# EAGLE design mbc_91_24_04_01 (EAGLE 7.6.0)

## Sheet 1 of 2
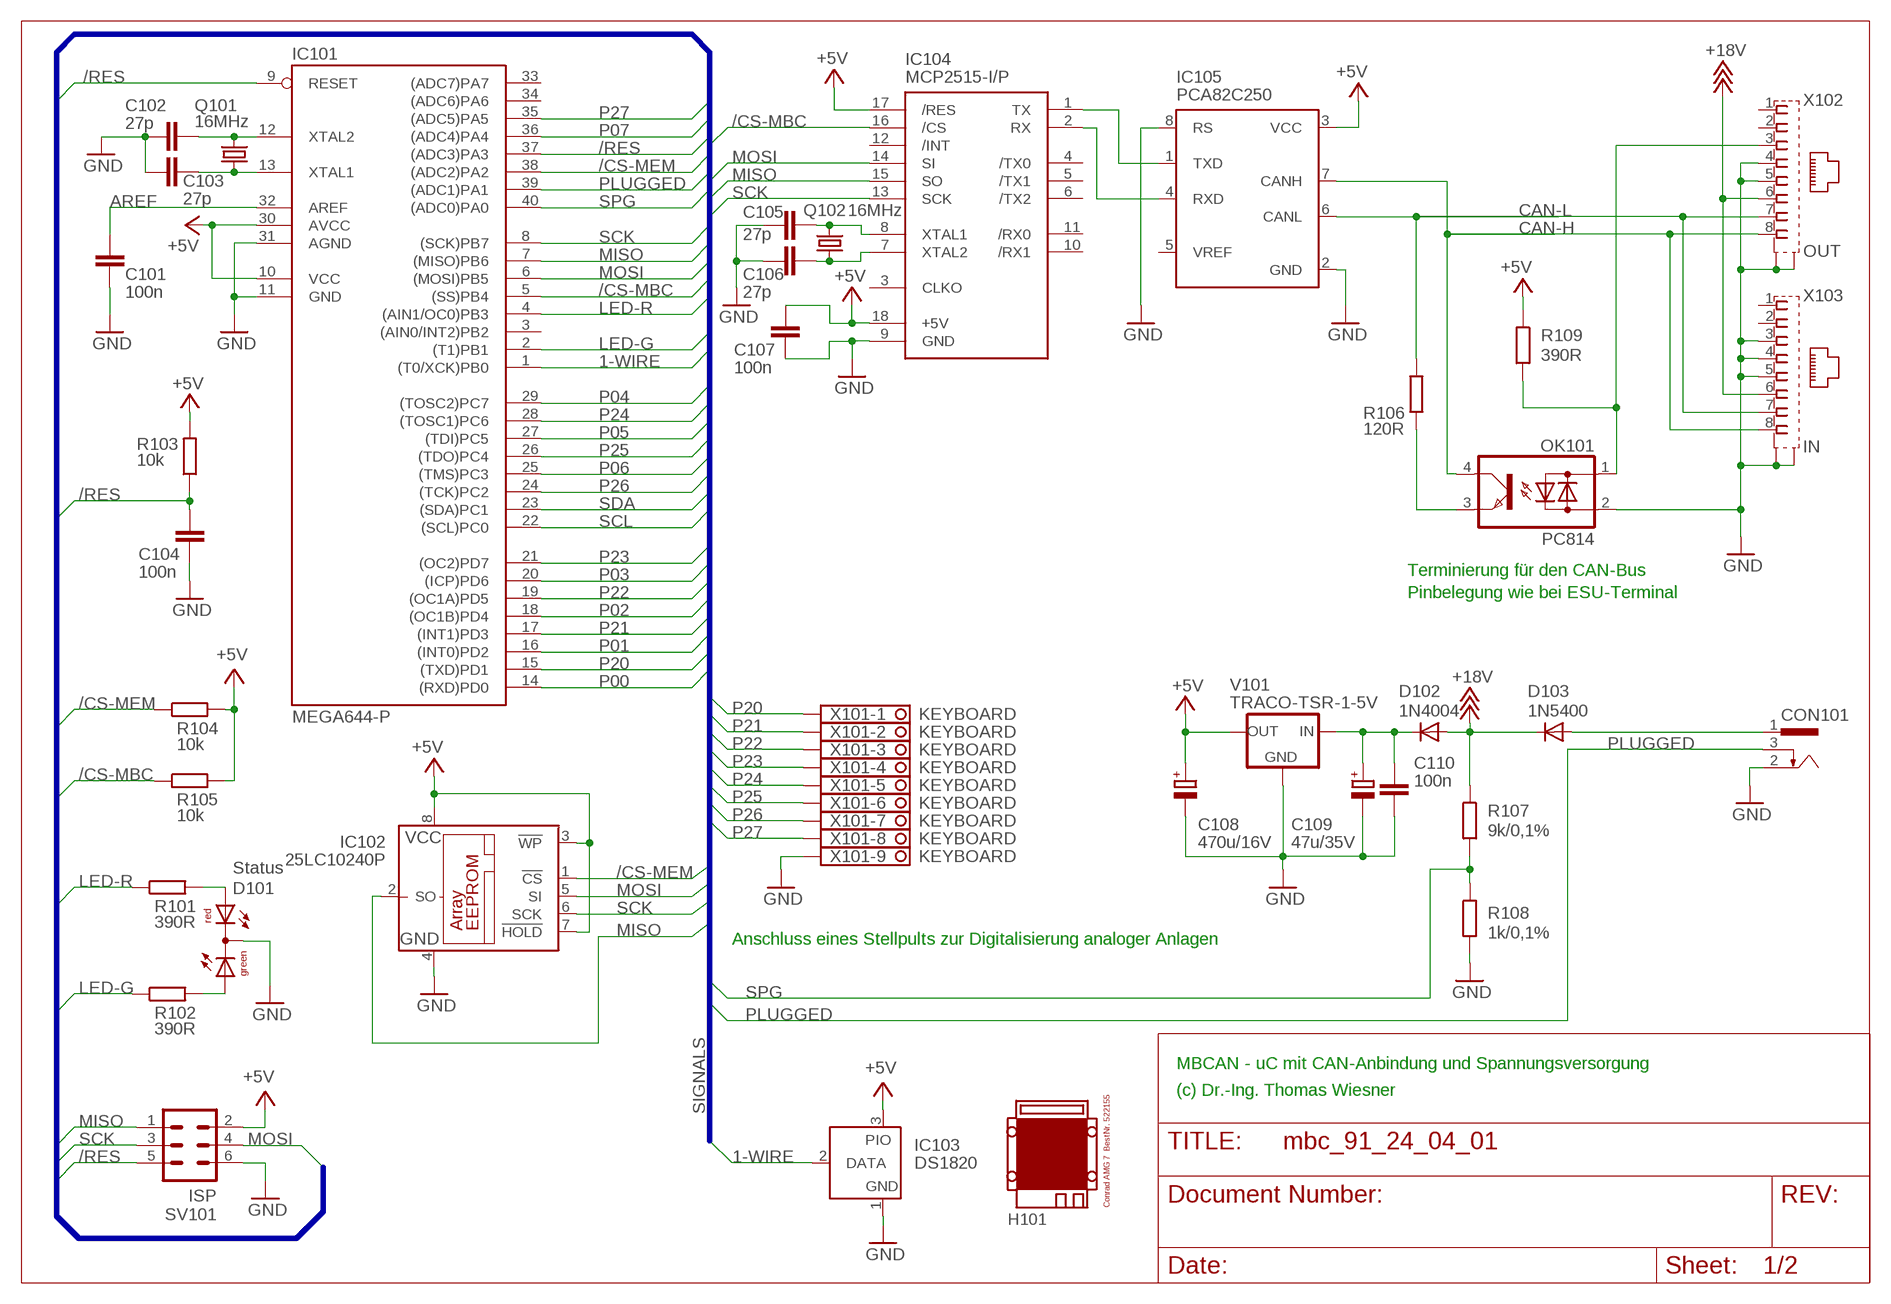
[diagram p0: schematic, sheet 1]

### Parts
C101  100n  C-EU025-025X050  [C025-025X050]
C102  27p  C-EU025-025X050  [C025-025X050]
C103  27p  C-EU025-025X050  [C025-025X050]
C104  100n  C-EU025-025X050  [C025-025X050]
C105  27p  C-EU025-025X050  [C025-025X050]
C106  27p  C-EU025-025X050  [C025-025X050]
C107  100n  C-EU025-025X050  [C025-025X050]
C108  470u/16V  CPOL-EUE3.5-8  [E3,5-8]
C109  47u/35V  CPOL-EUE2.5-7  [E2,5-7]
C110  100n  C-EU025-025X050  [C025-025X050]
CON101  POWER-JACK  [POWER-JACK]
D101  Status  DUOLED5MM  [DUOLED5MM]
D102  1N4004  [DO41-10]
D103  1N5400  [DO201-15]
H101  MODULGEHÄUSE-AMG-7  [MODULGEHÄUSE-AMG-7]
IC101  MEGA644-P  MEGA323-P  [DIL40]
IC102  25LC10240P  25LC040P  [DIL8]
IC103  DS1820  DS2405  [TO92-]
IC104  MCP2515-I/P  MCP2510-I/P  [DIL18]
IC105  PCA82C250  [DIL08]
OK101  PC814  [DIL04]
Q101  16MHz  CRYSTALHC49U70  [HC49U70]
Q102  16MHz  CRYSTALHC49U70  [HC49U70]
R101  390R  R-EU_0207/10  [0207/10]
R102  390R  R-EU_0207/10  [0207/10]
R103  10k  R-EU_0207/10  [0207/10]
R104  10k  R-EU_0207/10  [0207/10]
R105  10k  R-EU_0207/10  [0207/10]
R106  120R  R-EU_0207/10  [0207/10]
R107  9k/0,1%  R-EU_0207/10  [0207/10]
R108  1k/0,1%  R-EU_0207/10  [0207/10]
R109  390R  R-EU_0207/10  [0207/10]
SV101  ISP  ML6  [ML6]
V101  TRACO-TSR-1-5V  [TRACO-TSR-1]
X101  KEYBOARD  1751316  [1751316]
X102  OUT  0446200002  [0446200002]
X103  IN  0446200002  [0446200002]

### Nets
1-WIRE: IC101.1((T0/XCK)PB0) IC103.2(DATA)
+5V: C107.1 C108.+ IC101.10(VCC) IC101.30(AVCC) IC102.3(!WP) IC102.7(!HOLD) IC102.8(VCC) IC103.3(PIO) IC104.17(/RES) IC104.18(+5V) IC105.3(VCC) R103.2 R104.2 R105.2 R109.1 SV101.2 V101.OUT ; also sheet 2
+18V: D102.A D103.C R107.1 X102.6 X103.6 ; also sheet 2
/CS-MBC: IC101.5((SS)PB4) IC104.16(/CS) R105.1
/CS-MEM: IC101.38((ADC2)PA2) IC102.1(!CS) R104.1
/RES: C104.1 IC101.9(RESET) IC101.37((ADC3)PA3) R103.1 SV101.5
AREF: C101.1 IC101.32(AREF)
CAN-H: IC105.7(CANH) OK101.4(C) X102.8 X103.8
CAN-L: IC105.6(CANL) R106.2 X102.7 X103.7
GND: C101.2 C102.1 C103.1 C104.2 C105.1 C106.1 C107.2 C108.- C109.- C110.2 CON101.2 D101.K(C) IC101.11(GND) IC101.31(AGND) IC102.4(GND) IC103.1(GND) IC104.9(GND) IC105.2(GND) IC105.8(RS) OK101.2(AC2) R108.2 SV101.6 V101.GND X101.9 X102.4 X102.5 X102.S@1(S1) X102.S@2(S2) X103.3 X103.4 X103.5 X103.S@1(S1) X103.S@2(S2) ; also sheet 2
LED-G: IC101.2((T1)PB1) R102.1
LED-R: IC101.4((AIN1/OC0)PB3) R101.1
MISO: IC101.7((MISO)PB6) IC102.2(SO) IC104.15(SO) SV101.1
MOSI: IC101.6((MOSI)PB5) IC102.5(SI) IC104.14(SI) SV101.4
N$1: IC104.1(TX) IC105.1(TXD)
N$2: IC104.2(RX) IC105.4(RXD)
N$3: OK101.3(E) R106.1
N$4: OK101.1(AC1) R109.2 X102.3
N$6: C109.+ C110.1 D102.C V101.IN
N$9: D101.AR R101.2
N$13: D101.AG R102.2
N$21: C102.2 IC101.12(XTAL2) Q101.2
N$22: C103.2 IC101.13(XTAL1) Q101.1
N$23: C105.2 IC104.8(XTAL1) Q102.2
N$24: C106.2 IC104.7(XTAL2) Q102.1
P00: IC101.14((RXD)PD0) ; also sheet 2
P01: IC101.16((INT0)PD2) ; also sheet 2
P02: IC101.18((OC1B)PD4) ; also sheet 2
P03: IC101.20((ICP)PD6) ; also sheet 2
P04: IC101.29((TOSC2)PC7) ; also sheet 2
P05: IC101.27((TDI)PC5) ; also sheet 2
P06: IC101.25((TMS)PC3) ; also sheet 2
P07: IC101.36((ADC4)PA4) ; also sheet 2
P20: IC101.15((TXD)PD1) X101.1
P21: IC101.17((INT1)PD3) X101.2
P22: IC101.19((OC1A)PD5) X101.3
P23: IC101.21((OC2)PD7) X101.4
P24: IC101.28((TOSC1)PC6) X101.5
P25: IC101.26((TDO)PC4) X101.6
P26: IC101.24((TCK)PC2) X101.7
P27: IC101.35((ADC5)PA5) X101.8
PLUGGED: CON101.3 IC101.39((ADC1)PA1)
SCK: IC101.8((SCK)PB7) IC102.6(SCK) IC104.13(SCK) SV101.3
SCL: IC101.22((SCL)PC0) ; also sheet 2
SDA: IC101.23((SDA)PC1) ; also sheet 2
SPG: IC101.40((ADC0)PA0) R107.2 R108.1
V-NETZTEIL: CON101.1 D103.A
Unconnected: IC101.3((AIN0/INT2)PB2) IC101.33((ADC7)PA7) IC101.34((ADC6)PA6) IC104.3(CLKO) IC104.4(/TX0) IC104.5(/TX1) IC104.6(/TX2) IC104.10(/RX1) IC104.11(/RX0) IC104.12(/INT) IC105.5(VREF) X102.1 X102.2 X103.1 X103.2

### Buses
SIGNALS

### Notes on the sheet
- Terminierung für den CAN-Bus
- Pinbelegung wie bei ESU-Terminal
- Anschluss eines Stellpults zur Digitalisierung analoger Anlagen
- MBCAN - uC mit CAN-Anbindung und Spannungsversorgung
- (c) Dr.-Ing. Thomas Wiesner

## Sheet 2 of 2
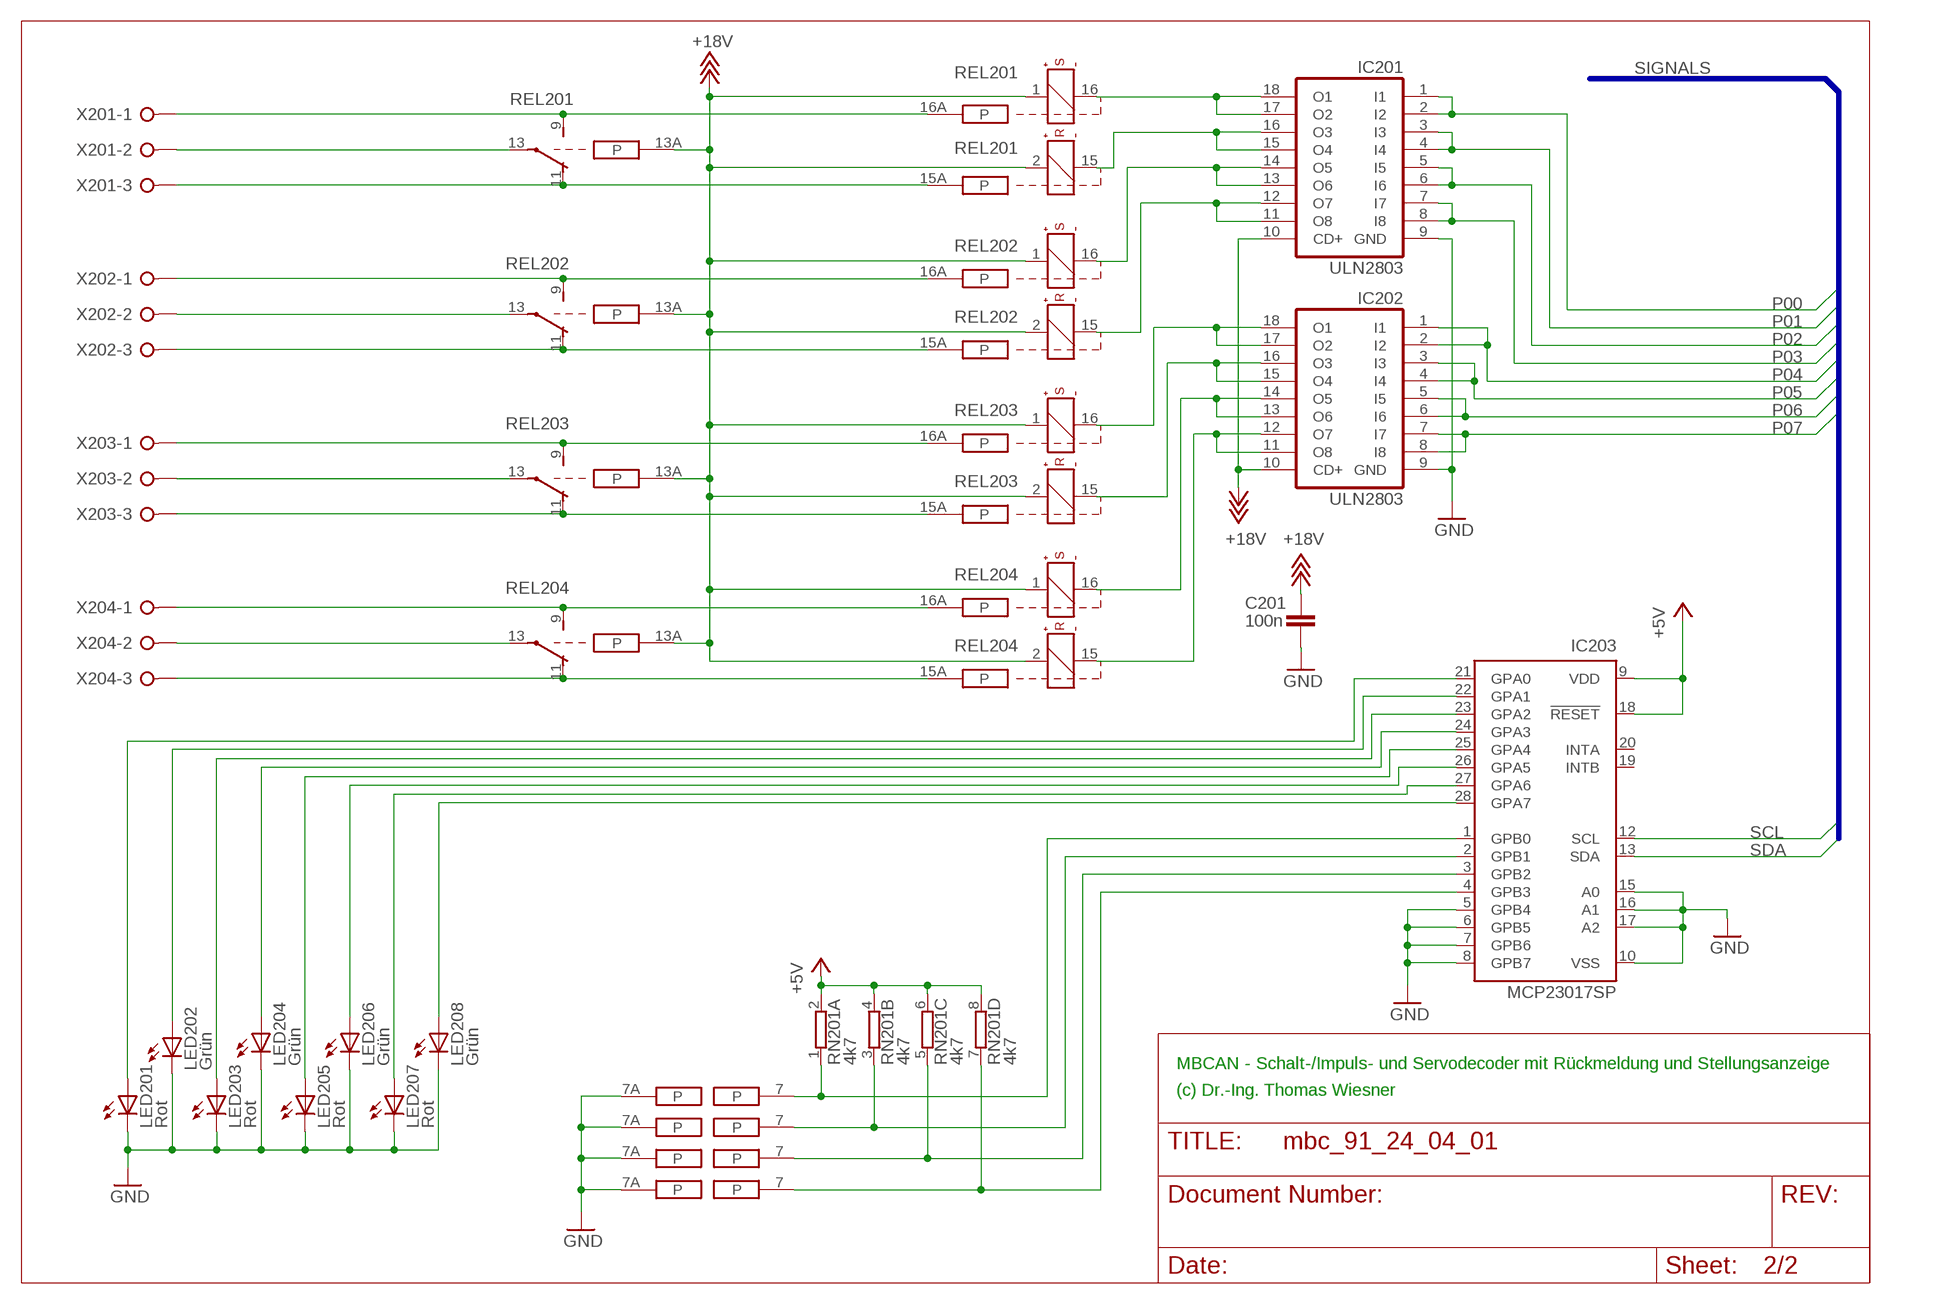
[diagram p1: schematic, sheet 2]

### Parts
C201  100n  C-EU025-025X050  [C025-025X050]
IC201  ULN2803  ULN2803A  [DIL18]
IC202  ULN2803  ULN2803A  [DIL18]
IC203  MCP23017SP  [DIL28-3]
LED201  Rot  LED3MM  [LED3MM]
LED202  Grün  LED3MM  [LED3MM]
LED203  Rot  LED3MM  [LED3MM]
LED204  Grün  LED3MM  [LED3MM]
LED205  Rot  LED3MM  [LED3MM]
LED206  Grün  LED3MM  [LED3MM]
LED207  Rot  LED3MM  [LED3MM]
LED208  Grün  LED3MM  [LED3MM]
REL201  RELAIS+PADS  [REL-BIPOLAR-LOETPADS]
REL202  RELAIS+PADS  [REL-BIPOLAR-LOETPADS]
REL203  RELAIS+PADS  [REL-BIPOLAR-LOETPADS]
REL204  RELAIS+PADS  [REL-BIPOLAR-LOETPADS]
RN201  4k7  E4R  [SIL8]
X201  W237-03P  [W237-133]
X202  W237-03P  [W237-133]
X203  W237-03P  [W237-133]
X204  W237-03P  [W237-133]

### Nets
+5V: IC203.9(VDD) IC203.18(!RESET) RN201.2 RN201.4 RN201.6 RN201.8 ; also sheet 1
+18V: C201.1 IC201.10(CD+) IC202.10(CD+) REL201.1(+) REL201.2(+) REL201.13A(P) REL202.1(+) REL202.2(+) REL202.13A(P) REL203.1(+) REL203.2(+) REL203.13A(P) REL204.1(+) REL204.2(+) REL204.13A(P) ; also sheet 1
GND: C201.2 IC201.9(GND) IC202.9(GND) IC203.5(GPB4) IC203.6(GPB5) IC203.7(GPB6) IC203.8(GPB7) IC203.10(VSS) IC203.15(A0) IC203.16(A1) IC203.17(A2) LED201.K(C) LED202.K(C) LED203.K(C) LED204.K(C) LED205.K(C) LED206.K(C) LED207.K(C) LED208.K(C) REL201.7A(P) REL202.7A(P) REL203.7A(P) REL204.7A(P) ; also sheet 1
K11: REL201.9(S) REL201.16A(P) X201.1
K12: REL201.13(P) X201.2
K13: REL201.11(O) REL201.15A(P) X201.3
K21: REL202.9(S) REL202.16A(P) X202.1
K22: REL202.13(P) X202.2
K23: REL202.11(O) REL202.15A(P) X202.3
K31: REL203.9(S) REL203.16A(P) X203.1
K32: REL203.13(P) X203.2
K33: REL203.11(O) REL203.15A(P) X203.3
K41: REL204.9(S) REL204.16A(P) X204.1
K42: REL204.13(P) X204.2
K43: REL204.11(O) REL204.15A(P) X204.3
N$5: IC203.22(GPA1) LED202.A
N$7: IC203.21(GPA0) LED201.A
N$8: IC201.15(O4) IC201.16(O3) REL201.15(-)
N$10: IC203.23(GPA2) LED203.A
N$11: IC203.25(GPA4) LED205.A
N$12: IC203.27(GPA6) LED207.A
N$14: IC203.1(GPB0) REL201.7(P) RN201.1
N$15: IC203.2(GPB1) REL202.7(P) RN201.3
N$16: IC203.3(GPB2) REL203.7(P) RN201.5
N$17: IC203.4(GPB3) REL204.7(P) RN201.7
N$18: IC203.24(GPA3) LED204.A
N$19: IC203.26(GPA5) LED206.A
N$20: IC203.28(GPA7) LED208.A
N$37: IC201.11(O8) IC201.12(O7) REL202.15(-)
N$50: IC202.15(O4) IC202.16(O3) REL203.15(-)
N$52: IC202.11(O8) IC202.12(O7) REL204.15(-)
P00: IC201.1(I1) IC201.2(I2) ; also sheet 1
P01: IC201.3(I3) IC201.4(I4) ; also sheet 1
P02: IC201.5(I5) IC201.6(I6) ; also sheet 1
P03: IC201.7(I7) IC201.8(I8) ; also sheet 1
P04: IC202.1(I1) IC202.2(I2) ; also sheet 1
P05: IC202.3(I3) IC202.4(I4) ; also sheet 1
P06: IC202.5(I5) IC202.6(I6) ; also sheet 1
P07: IC202.7(I7) IC202.8(I8) ; also sheet 1
S1: IC201.17(O2) IC201.18(O1) REL201.16(-)
S2: IC201.13(O6) IC201.14(O5) REL202.16(-)
S3: IC202.17(O2) IC202.18(O1) REL203.16(-)
S4: IC202.13(O6) IC202.14(O5) REL204.16(-)
SCL: IC203.12(SCL) ; also sheet 1
SDA: IC203.13(SDA) ; also sheet 1
Unconnected: IC203.19(INTB) IC203.20(INTA) REL201.4(P) REL201.6(O) REL201.8(S) REL202.4(P) REL202.6(O) REL202.8(S) REL203.4(P) REL203.6(O) REL203.8(S) REL204.4(P) REL204.6(O) REL204.8(S)

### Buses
SIGNALS

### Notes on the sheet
- MBCAN - Schalt-/Impuls- und Servodecoder mit Rückmeldung und Stellungsanzeige
- (c) Dr.-Ing. Thomas Wiesner

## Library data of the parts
C101-C107 C110 C201 = rcl:C-EU: CAPACITOR, European symbol
C108 C109 = rcl:CPOL-EU: POLARIZED CAPACITOR, European symbol
CON101 = mbc:POWER-JACK: Power-Stecker für 2,5 mm Hohlbuchse
D101 = led:DUOLED5MM: DUO LED 2 colors, 5 mm, round
D102 = diode:1N4004: DIODE
D103 = diode:1N5400: DIODE
H101 = mbc:MODULGEHÄUSE-AMG-7: Gehäuse
IC101 = atmel:MEGA323-P: MICROCONTROLLER 32 Kbytes FLASH 2 Kbytes SRAM 1 Kbytes EEPROM USART 8-channel 10 bit ADC Source: avr.lbr; OC_FARNELL: unknown; OC_NEWARK: unknown
IC102 = microchip:25*: Serial EEPROM 4K/ 8K , SPI bus; MF: MICROCHIP; MPN: 25LC040/P; OC_FARNELL: 9758100; OC_NEWARK: 96K4091
IC103 = maxim:DS2405: Addressable Switch DALLAS Semiconductor; MF: DALLAS SEMICONDUCTOR; MPN: DS2405; OC_FARNELL: 1188025; OC_NEWARK: 06F4645
IC104 = mbc:MCP2510: BASIC-CAN 2.0a Controller Stand-alone CAN controller von Microchip
IC105 = micro-philips:PCA82C250: CAN CONTROLLER INTERFACE; OC_FARNELL: 3692358; OC_NEWARK: unknown
IC201 IC202 = uln-udn:ULN2803A: DRIVER ARRAY
IC203 = microchip:MCP23017: http://ww1.microchip.com/downloads/en/DeviceDoc/21952a.pdf Source: http://ww1.microchip.com/downloads/en/DeviceDoc/21952a.pdf; MF: MICROCHIP; MPN: MCP23017-E/SP; OC_FARNELL: 1332088; OC_NEWARK: 31K2959
LED201-LED208 = led:LED: LED
OK101 = optocoupler:PC814: SHARP OPTO COUPLER; OC_FARNELL: 9707662; OC_NEWARK: unknown
Q101 Q102 = crystal:CRYSTAL: CRYSTAL; OC_FARNELL: unknown; OC_NEWARK: unknown
R101-R109 = resistor:R-EU_: RESISTOR, European symbol
REL201-REL204 = mbc:RELAIS+PADS: Bistabiles Relais 2xUM 12V mit Lötbrücken
RN201 = resistor-sil:E4R: SIL RESISTOR; OC_FARNELL: unknown; OC_NEWARK: unknown
SV101 = con-ml:ML6: HARTING; OC_FARNELL: unknown; OC_NEWARK: unknown
V101 = mbc:TRACO-TSR-1-5V: Spannungsregler Hersteller: TRACO Typ: TSR-1 5V: TSR 1-2450 Spg: 5V Strom: 1A Reichelt TSR 1-2450
X101 = con-phoenix-350:1751316: MKDS 1/ 9-3,5 Printklemme Nennstrom: 10 A Bemessungsspannung: 160 V Raster: 3,5 mm Polzahl: 9 Montageart: Löten Anschlussart: Schraubanschluss Anschlussrichtung vom Leiter zur Platine: 0° Source: http://eshop.phoenixcontact.com .. 1751316.pdf; OC_FARNELL: unknown; OC_NEWARK: unknown
X102 X103 = mbc:0446200002: RJ-45 INVERTED MODULAR JACK ASSEMBLY WITH RJ-11 KEEPOUT FEATURE Source: Data sheet MOLEX 0446200002 BUCHSE, RJ45, GESCHIRMT Source: Farnell; MF: MOLEX; MPN: 0446200002; OC_FARNELL: 9251910
X201-X204 = con-wago-508:W237-03P: WAGO SREW CLAMP; OC_FARNELL: unknown; OC_NEWARK: unknown

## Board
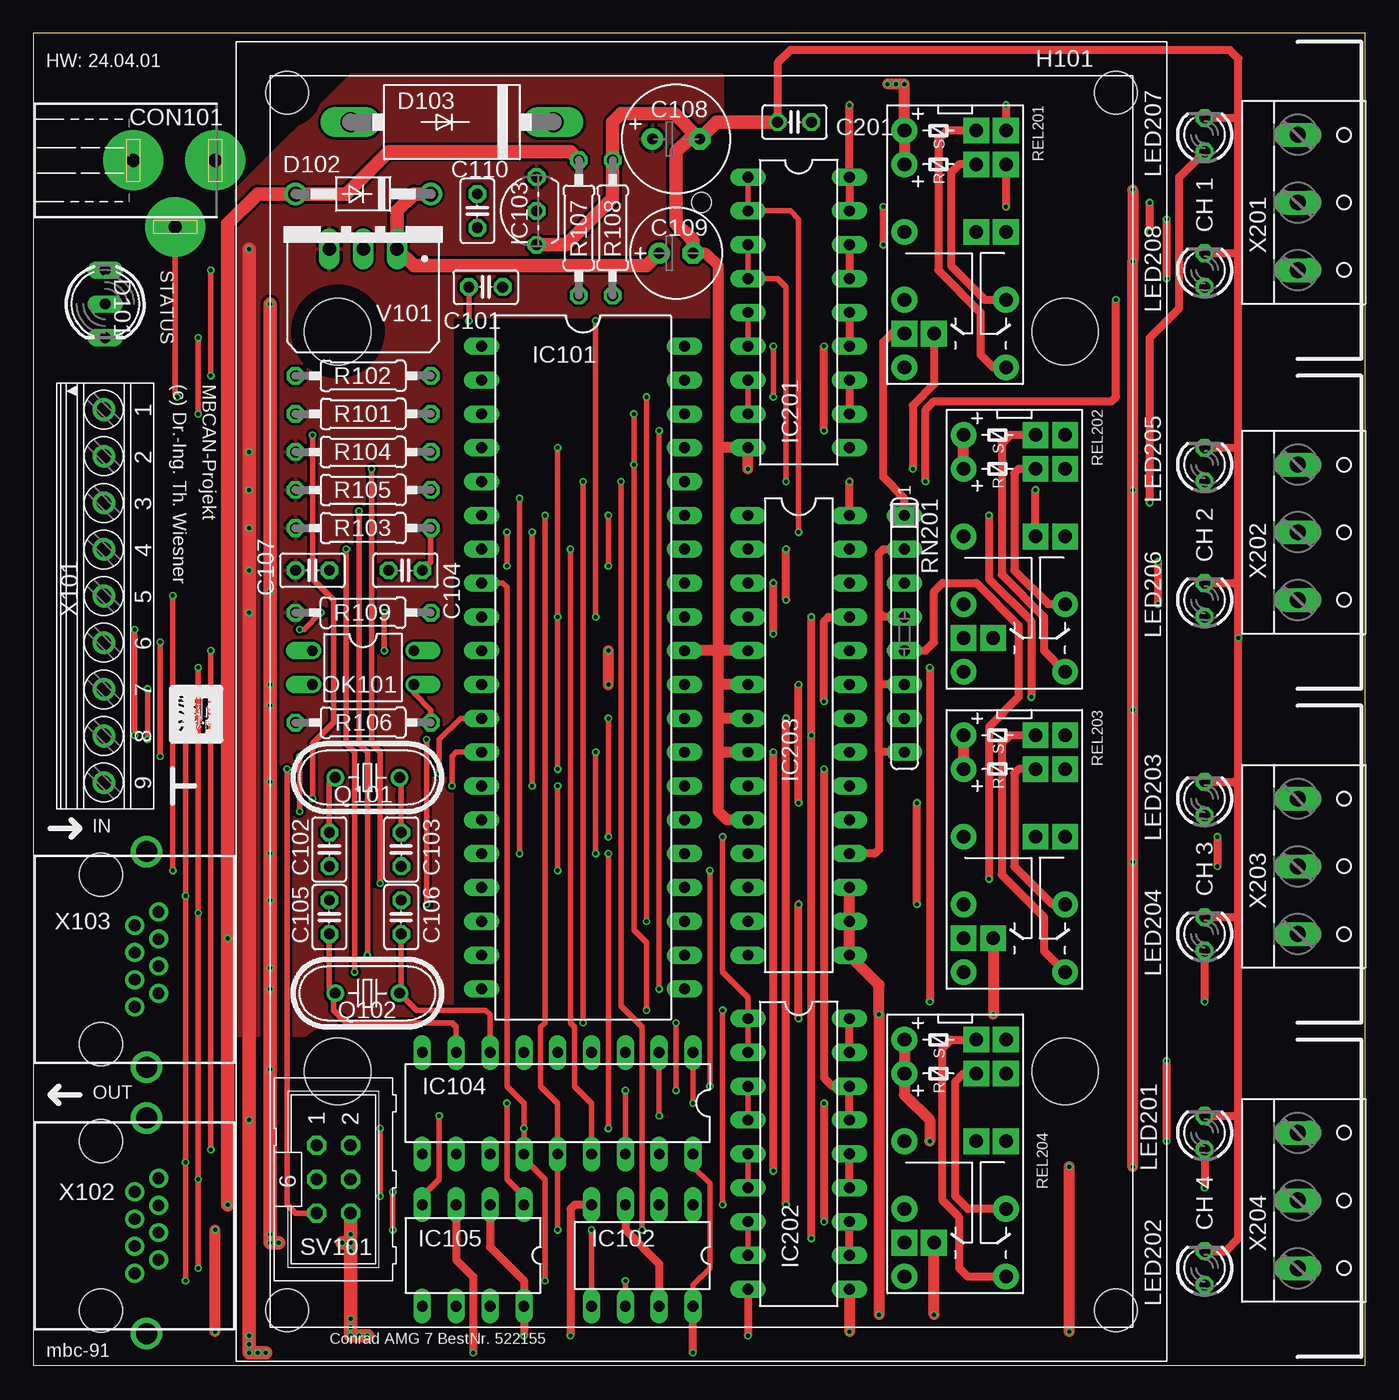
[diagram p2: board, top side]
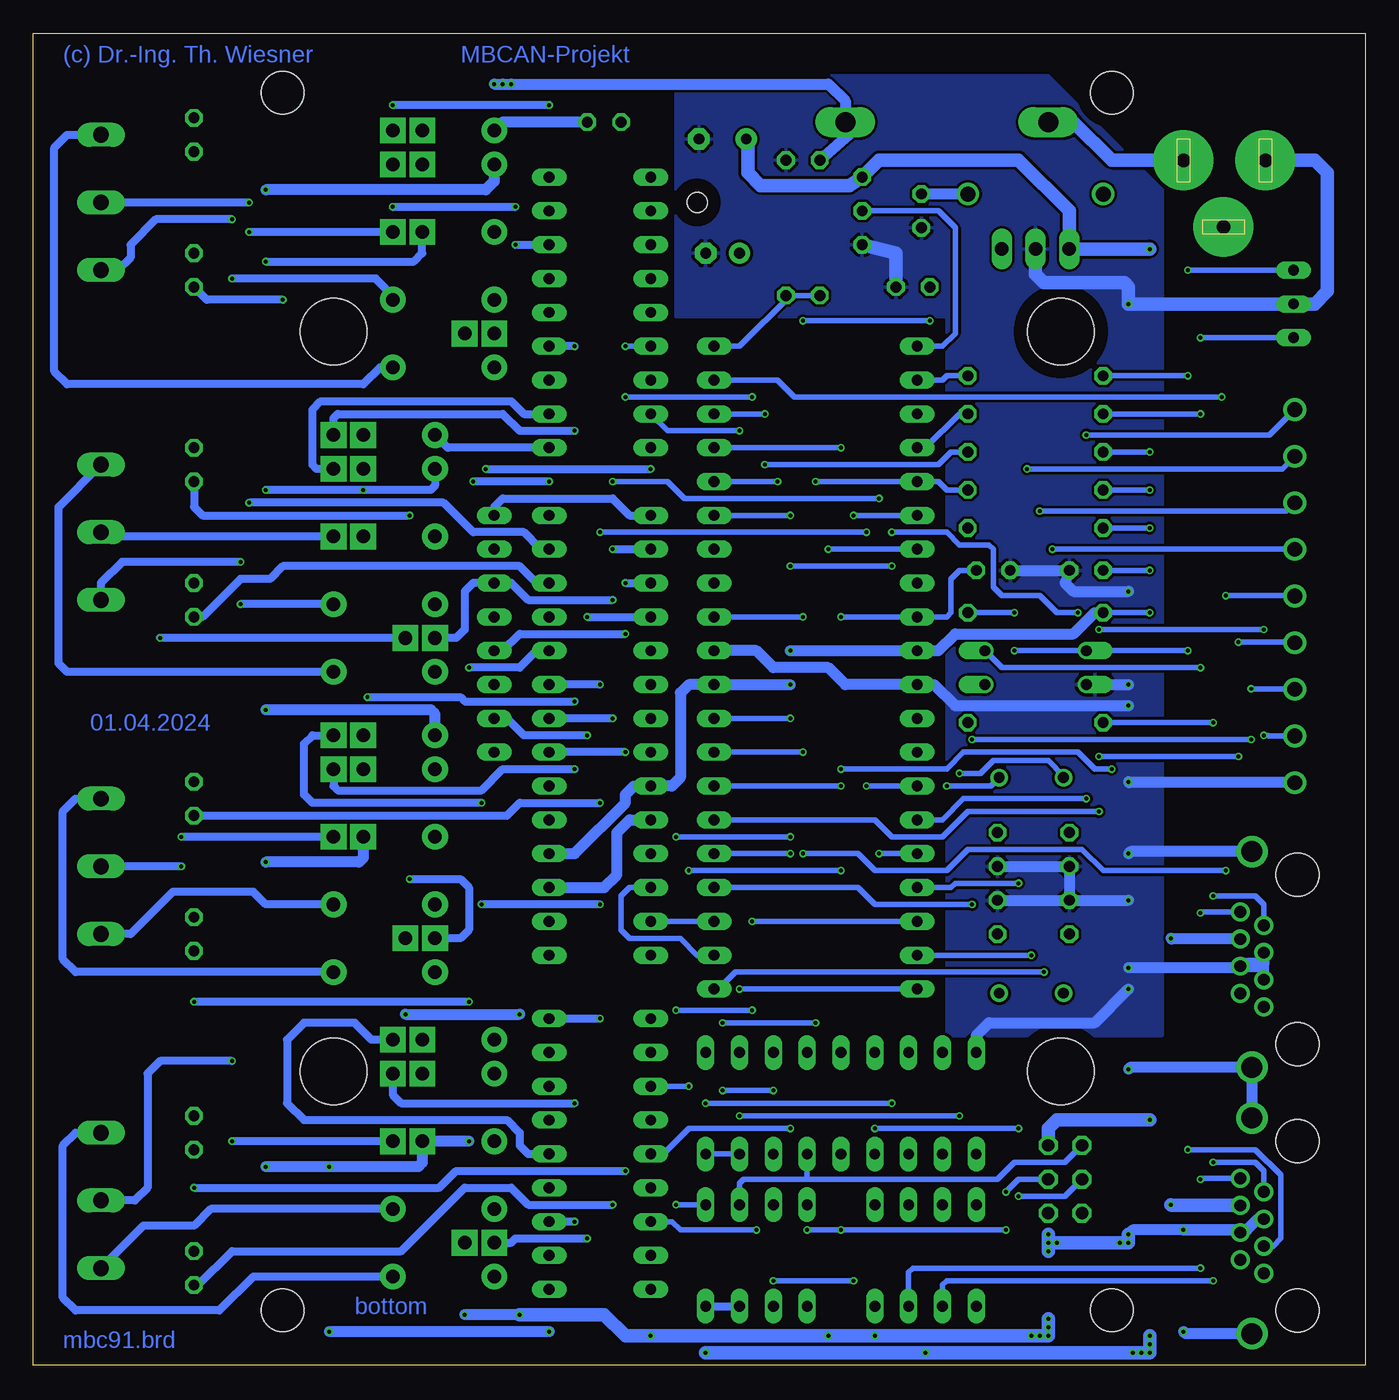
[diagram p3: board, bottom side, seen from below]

Size 100.01 x 100.01 mm. Coordinates in mm from the lower left corner, seen from the top.
Outline: 100,0.02 0,0.02 0,100.01 100,100.01
Outline: 100.01,0 100.01,100.01
Copper layers (1*16): Top 0.035mm / dielectric 1.5mm / Bottom 0.035mm
Design rules "default *": minimum track width 10mil, minimum drill 0.3mm, track to track 8mil, track to pad 8mil, pad to pad 8mil, via to via 8mil, smd to smd 8mil, copper to edge 40mil, drill to drill 8mil, minimum pad ring 10mil, minimum via ring 0.125mm, stop-mask expansion 4mil, vias tented up to drill 0mil, thermal gap 10mil

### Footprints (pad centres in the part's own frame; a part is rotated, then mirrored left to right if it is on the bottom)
C025-025X050 = drill 0.813 octagon: 1 -1.27,0; 2 1.27,0
E3,5-8 = drill 0.813 pad 1.6: + -1.778,0 | drill 0.813 pad 1.6 octagon: - 1.778,0
E2,5-7 = drill 0.813 pad 1.6: + -1.27,0 | drill 0.813 pad 1.6 octagon: - 1.27,0
POWER-JACK = drill 1 pad 4.5: 1 0,6.03; 2 0,-0.12; 3 5,3.03
DUOLED5MM = drill 0.813 long: AG -2.54,0; AR 2.54,0; K 0,0
DO41-10 = drill 1.118: A 5.08,0; C -5.08,0
DO201-15 = drill 1.499 long: A 7.62,0; C -7.62,0
MODULGEHÄUSE-AMG-7 = hole 3.2: -45.72,-31.115; -45.72,31.115; 45.72,31.115; 45.72,-31.115 | hole 5: -27.781,-27.305; 27.781,-27.305; -27.781,27.305; 27.781,27.305 | hole 1.5: -37.465,0
DIL40 = drill 0.813 long: 1 -24.13,-7.62; 2 -21.59,-7.62; 3 -19.05,-7.62; 4 -16.51,-7.62; 5 -13.97,-7.62; 6 -11.43,-7.62; 7 -8.89,-7.62; 8 -6.35,-7.62; 9 -3.81,-7.62; 10 -1.27,-7.62; 11 1.27,-7.62; 12 3.81,-7.62; 13 6.35,-7.62; 14 8.89,-7.62; 15 11.43,-7.62; 16 13.97,-7.62; 17 16.51,-7.62; 18 19.05,-7.62; 19 21.59,-7.62; 20 24.13,-7.62; 21 24.13,7.62; 22 21.59,7.62; 23 19.05,7.62; 24 16.51,7.62; 25 13.97,7.62; 26 11.43,7.62; 27 8.89,7.62; 28 6.35,7.62; 29 3.81,7.62; 30 1.27,7.62; 31 -1.27,7.62; 32 -3.81,7.62; 33 -6.35,7.62; 34 -8.89,7.62; 35 -11.43,7.62; 36 -13.97,7.62; 37 -16.51,7.62; 38 -19.05,7.62; 39 -21.59,7.62; 40 -24.13,7.62
DIL8 = drill 0.813 long: 1 -3.81,-3.81; 2 -1.27,-3.81; 3 1.27,-3.81; 4 3.81,-3.81; 5 3.81,3.81; 6 1.27,3.81; 7 -1.27,3.81; 8 -3.81,3.81
TO92- = drill 0.813 octagon: 1 -2.54,0; 2 0,0; 3 2.54,0
DIL18 = drill 0.813 long: 1 -10.16,-3.81; 2 -7.62,-3.81; 3 -5.08,-3.81; 4 -2.54,-3.81 | drill 0.8 long: 5 0,-3.81; 6 2.54,-3.81; 7 5.08,-3.81; 8 7.62,-3.81; 9 10.16,-3.81; 10 10.16,3.81; 11 7.62,3.81; 12 5.08,3.81; 13 2.54,3.81; 14 0,3.81; 15 -2.54,3.81; 16 -5.08,3.81; 17 -7.62,3.81; 18 -10.16,3.81
DIL08 = drill 0.813 long: 1 -3.81,-3.81; 2 -1.27,-3.81; 3 1.27,-3.81; 4 3.81,-3.81; 5 3.81,3.81; 6 1.27,3.81; 7 -1.27,3.81; 8 -3.81,3.81
DIL18' = drill 0.813 long: 1 -10.16,-3.81; 2 -7.62,-3.81; 3 -5.08,-3.81; 4 -2.54,-3.81; 5 0,-3.81; 6 2.54,-3.81; 7 5.08,-3.81; 8 7.62,-3.81; 9 10.16,-3.81; 10 10.16,3.81; 11 7.62,3.81; 12 5.08,3.81; 13 2.54,3.81; 14 0,3.81; 15 -2.54,3.81; 16 -5.08,3.81; 17 -7.62,3.81; 18 -10.16,3.81
DIL28-3 = drill 0.813 long: 1 -16.51,-3.81; 2 -13.97,-3.81; 3 -11.43,-3.81; 4 -8.89,-3.81; 5 -6.35,-3.81; 6 -3.81,-3.81; 7 -1.27,-3.81; 8 1.27,-3.81; 9 3.81,-3.81; 10 6.35,-3.81; 11 8.89,-3.81; 12 11.43,-3.81; 13 13.97,-3.81; 14 16.51,-3.81; 15 16.51,3.81; 16 13.97,3.81; 17 11.43,3.81; 18 8.89,3.81; 19 6.35,3.81; 20 3.81,3.81; 21 1.27,3.81; 22 -1.27,3.81; 23 -3.81,3.81; 24 -6.35,3.81; 25 -8.89,3.81; 26 -11.43,3.81; 27 -13.97,3.81; 28 -16.51,3.81
LED3MM = drill 0.813 octagon: A -1.27,0; K 1.27,0
DIL04 = drill 0.813 offset: 1 -1.27,-3.81; 2 1.27,-3.81; 3 1.27,3.81; 4 -1.27,3.81
HC49U70 = drill 0.813: 1 -2.413,0; 2 2.413,0
0207/10 = drill 0.813 octagon: 1 -5.08,0; 2 5.08,0
REL-BIPOLAR-LOETPADS = drill 1.016 pad 1.93: 1 -8.89,-3.81; 2 -6.35,-3.81; 4 -1.27,-3.81; 6 3.81,-3.81; 8 8.89,-3.81; 9 8.89,3.81; 11 3.81,3.81 | drill 1.016 pad 1.93 square: 7 6.35,-3.81; 7A 6.35,-1.587; 13 -1.27,3.81; 13A -1.27,1.587; 15 -6.35,3.81; 15A -6.35,1.587; 16 -8.89,3.81; 16A -8.89,1.587
SIL8 = drill 0.813 long: 1 -8.89,0; 2 -6.35,0; 3 -3.81,0; 4 -1.27,0; 5 1.27,0; 6 3.81,0; 7 6.35,0; 8 8.89,0
ML6 = drill 0.914 octagon: 1 -2.54,-1.27; 2 -2.54,1.27; 3 0,-1.27; 4 0,1.27; 5 2.54,-1.27; 6 2.54,1.27
TRACO-TSR-1 = drill 1.016 long: GND 0,2.54; IN -2.54,2.54; OUT 2.54,2.54
1751316 = drill 1.1 pad 1.7: 1 -13.973,-0.1; 2 -10.473,-0.1; 3 -6.973,-0.1; 4 -3.473,-0.1; 5 0.028,-0.1; 6 3.527,-0.1; 7 7.027,-0.1; 8 10.527,-0.1; 9 14.027,-0.1
0446200002 = drill 0.889 pad 1.422: 1 3.556,2.54; 2 2.54,4.318; 3 1.524,2.54; 4 0.508,4.318; 5 -0.508,2.54; 6 -1.524,4.318; 7 -2.54,2.54; 8 -3.556,4.318 | drill 1.575 pad 2.286: S@1 -8.103,3.429; S@2 8.103,3.429 | hole 3.251: 6.35,0; -6.35,0
W237-133 = drill 1.194 long: 1 -5.08,-0.635; 2 0,-0.635; 3 5.08,-0.635

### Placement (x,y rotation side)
C101  33.97,80.96 0 top
C102  22.23,38.73 90 top
C103  27.62,38.73 90 top
C104  27.94,59.69 180 top
C105  22.23,33.66 270 top
C106  27.62,33.66 270 top
C107  20.95,59.69 0 top
C108  48.26,92.08 0 top
C109  48.26,83.5 0 top
C110  33.34,86.68 270 top
C201  57.15,93.34 180 top
CON101  7.62,90.47 270 top
D101  5.4,79.69 270 top
D102  24.77,87.95 180 top
D103  31.43,93.34 180 top
H101  50.16,49.85 270 top
IC101  41.27,52.39 270 top
IC102  45.72,8.26 180 top
IC103  37.78,86.68 90 top
IC104  39.37,19.68 180 top
IC105  33.02,8.26 180 top
IC201  ULN2803  [DIL18']  57.47,79.06 270 top
IC202  ULN2803  [DIL18']  57.47,15.88 270 top
IC203  57.47,47.31 270 top
LED201  87.95,17.46 90 top
LED202  87.95,7.3 90 top
LED203  87.95,42.55 90 top
LED204  87.95,32.38 90 top
LED205  87.95,67.63 90 top
LED206  87.95,57.47 90 top
LED207  87.95,92.39 90 top
LED208  87.95,82.23 90 top
OK101  24.77,52.39 270 top
Q101  25.08,44.13 180 top
Q102  25.08,27.94 180 top
R101  24.77,71.44 180 top
R102  24.77,74.3 180 top
R103  24.77,62.87 180 top
R104  24.77,68.58 180 top
R105  24.77,65.72 180 top
R106  24.77,48.26 180 top
R107  40.96,85.41 270 top
R108  43.5,85.41 90 top
R109  24.77,56.52 0 top
REL201  69.22,83.82 270 top
REL202  73.66,60.96 270 top
REL203  73.66,38.42 270 top
REL204  69.22,15.56 270 top
RN201  65.41,54.93 270 top
SV101  22.54,13.97 270 top
V101  24.77,86.36 180 top
X101  5.4,57.78 270 top
X102  5.08,10.48 270 top
X103  5.08,30.48 270 top
X201  95.57,87.31 270 top
X202  95.57,62.55 270 top
X203  95.57,37.47 270 top
X204  95.57,12.38 270 top

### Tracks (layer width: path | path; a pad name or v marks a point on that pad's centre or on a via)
1-WIRE
  Bottom 0.406: IC103.2 32.07,86.68 30.8,85.41 30.8,77.47 31.75,76.52 IC101.1
+5V  (via drill 0.3)
  Top 0.406: IC104.18 49.53,14.92 50.8,13.65 50.8,7.3 49.53,6.03 IC102.8
  Top 0.61: RN201.8 63.5,46.04 | 63.5,46.04 63.5,51.12 | 63.5,51.12 63.5,56.52 | 63.5,56.52 63.5,60.96 63.82,61.28 RN201.2 | RN201.4 63.82,56.2 63.5,56.52 | RN201.6 63.5,51.12 | 63.5,46.04 63.5,38.73 63.18,38.42 IC203.18 | v49.53,0.95 IC102.8 | IC105.3 31.75,7.94 33.02,6.67 v33.02,0.95 | IC102.3 44.45,10.16 46.99,7.62 IC102.7
  Top 0.813: v43.18,51.12 v43.18,53.66
  Top 1.016: v16.19,83.82 v16.19,68.58 v16.19,65.72 v16.19,62.87 v16.19,59.69 v16.19,56.52 v16.19,18.41 v16.19,2.22 v16.19,1.59 v16.19,0.95 v16.83,0.95 v17.46,0.95
  Bottom 0.406: R104.2 v16.19,68.58 | R105.2 v16.19,65.72 | R103.2 v16.19,62.87 | C107.1 v16.19,59.69 | R109.1 v16.19,56.52 | IC104.17 IC104.18
  Bottom 0.61: IC102.8 IC102.7
  Bottom 0.813: IC203.18 59.37,38.42 55.56,42.23 55.56,42.86 54.93,43.5 IC203.9 52.07,43.5 51.44,44.13 51.44,50.48 50.8,51.12 IC101.30 v43.18,51.12 | v43.18,53.66 IC101.10 32.07,53.66 30.8,54.93 21.91,54.93 20.32,56.52 R109.1
  Bottom 1.016: v16.19,83.82 V101.OUT 22.23,86.68 26.04,90.49 36.51,90.49 IC103.3 38.73,88.58 45.4,88.58 46.35,89.53 46.35,91.95 C108.+ | v49.53,0.95 v33.02,0.95 v17.46,0.95 v16.83,0.95 v16.19,0.95 v16.19,1.59 v16.19,2.22 | SV101.2 23.81,17.78 23.18,18.41 v16.19,18.41
  pour Top: 15.24,24.77 15.24,88.27 23.81,96.84 51.75,96.84 51.75,78.74 31.43,78.74 31.43,24.77
+18V  (via drill 0.3)
  Top 0.61: REL202.13A v75.25,65.72
  Top 0.813: REL201.2 REL201.1 v65.41,96.2 v64.77,96.2 v64.14,96.2 | REL202.2 REL202.1 | REL203.1 REL203.2 | REL204.1 REL204.2 65.41,20.32 67.31,18.41 v67.31,16.83 | v82.55,14.92 v82.55,37.78 v82.55,49.21 v82.55,65.72 v82.55,82.87 v82.55,88.27 | IC202.10 v61.28,2.54 | v77.79,2.54 v77.79,14.92
  Top 1.016: v14.61,12.06 v14.61,32.07 14.61,85.72 16.83,87.95 D102.A 23.5,87.95 26.67,91.12 40.32,91.12 R107.1
  Bottom 0.61: v82.55,82.87 71.44,82.87 70.8,83.5 REL201.13A | REL202.2 69.85,66.04 70.17,65.72 v75.25,65.72 v82.55,65.72 | IC201.10 68.9,68.9 REL202.1
  Bottom 0.813: v82.55,14.92 v77.79,14.92 71.12,14.92 70.8,15.24 REL204.13A v67.31,16.83 | REL201.2 65.41,88.9 66.04,88.27 v82.55,88.27 | REL203.1 69.85,48.9 70.17,49.21 v82.55,49.21 | REL203.13A 75.25,38.1 75.56,37.78 v82.55,37.78 | v61.28,2.54 v77.79,2.54 | X103.6 14.54,32 v14.61,32.07 | v65.41,96.2 v64.77,96.2 v64.14,96.2 40.32,96.2 39.05,94.93 D103.C 38.42,92.71 R107.1 | C201.1 64.77,93.34 REL201.1
  Bottom 1.016: X102.6 14.54,12 v14.61,12.06
/CS-MBC  (via drill 0.3)
  Top 0.406: IC104.16 v44.45,20.64 | v48.26,20.64 v48.26,25.72 | v41.27,25.72 v41.27,66.36
  Bottom 0.406: v44.45,20.64 v48.26,20.64 | v48.26,25.72 v41.27,25.72 | v41.27,66.36 IC101.5 32.07,66.36 31.43,65.72 R105.1
/CS-MEM  (via drill 0.3)
  Top 0.406: v45.09,71.44 v45.09,67.63 45.09,32.7 46.04,31.75 v46.04,26.67 | v51.75,26.67 v51.75,12.06
  Bottom 0.406: R104.1 31.11,68.58 32.07,67.63 v45.09,67.63 | v45.09,71.44 IC101.38 | v46.04,26.67 v51.75,26.67 | v51.75,12.06 IC102.1
/RES  (via drill 0.3)
  Top 0.406: SV101.5 19.68,11.43 19.05,12.06 v19.05,44.77 | v39.37,44.77 v39.37,56.2 v39.37,68.9 | R103.1 29.84,60.33 C104.1
  Bottom 0.406: v19.05,44.77 20.32,44.77 21.59,46.04 30.16,46.04 31.43,44.77 v39.37,44.77 | v39.37,56.2 IC101.9 31.43,56.2 31.11,56.52 31.11,59.05 30.48,59.69 C104.1 | IC101.37 v39.37,68.9
AREF  (via drill 0.3)
  Top 0.406: v42.23,56.2 v42.23,78.42 | v32.7,78.42 C101.1
  Bottom 0.406: IC101.32 v42.23,56.2 | v42.23,78.42 v32.7,78.42
CAN-H  (via drill 0.3)
  Top 0.406: v12.38,7.3 v12.38,13.97 v12.38,33.97 v12.38,52.39
  Bottom 0.406: IC105.7 34.29,6.99 33.97,7.3 v12.38,7.3 | v12.38,52.39 27.3,52.39 OK101.4 | X102.8 12.32,14.03 v12.38,13.97 | X103.8 12.32,34.04 v12.38,33.97
CAN-L  (via drill 0.3)
  Top 0.406: v11.43,6.35 v11.43,15.24 v11.43,35.24 v11.43,48.26
  Bottom 0.406: IC105.6 31.75,6.03 31.43,6.35 v11.43,6.35 | v11.43,48.26 R106.2 | X102.7 7.62,14.61 8.26,15.24 v11.43,15.24 | X103.7 7.62,34.61 8.26,35.24 v11.43,35.24
GND  (via drill 0.3)
  Top 0.61: LED202.K 89.53,8.57 90.49,9.53 90.49,18.73 | 90.49,18.73 90.49,33.34 | 90.49,33.34 90.49,43.5 | 90.49,43.5 v90.49,54.61 90.49,58.42 | 90.49,58.42 90.49,68.9 | 90.49,68.9 90.49,83.5 | 90.49,83.5 90.49,93.66 | 90.49,93.66 90.49,98.11 89.85,98.74 56.83,98.74 55.88,97.79 C201.2 | LED207.K 90.49,93.66 | LED208.K 90.49,83.5 | LED205.K 90.49,68.9 | LED206.K 90.17,58.74 90.49,58.42 | LED203.K 90.17,43.81 90.49,43.5 | LED204.K 90.17,33.66 90.49,33.34 | LED201.K 90.49,18.73 | REL201.7A 67.63,73.66 66.04,72.07 v66.04,67.31 | IC202.9 v53.66,2.22 | v36.83,2.22 IC105.8 36.83,6.35 34.29,8.89 IC105.2 | IC102.4 40.64,12.06 40.32,11.75 v40.32,2.22
  Top 0.813: v63.5,3.81 v63.5,26.35 63.5,28.57 IC203.15 IC203.16 IC203.17 | v67.63,3.81 REL204.7A | REL203.7A v72.07,26.35 | IC203.10 52.07,40.96 51.44,41.59 51.44,46.04 | 51.44,46.04 51.44,48.58 | 51.44,48.58 51.44,51.12 | 51.44,51.12 51.44,53.66 | 51.44,53.66 51.44,68.9 | 51.44,68.9 51.44,82.55 50.48,83.5 C109.- | v53.66,67.31 IC201.9 51.44,68.9 | 51.44,46.04 IC203.8 | IC203.7 51.44,48.58 | IC203.6 51.44,51.12 | IC203.5 51.44,53.66 | 51.44,53.66 IC101.31 | v13.65,2.54 v13.65,10.16
  Top 1.016: v23.81,9.21 v23.81,8.57 v23.81,3.49 v23.81,2.86 v23.81,2.22 v25.08,2.22 | v23.81,9.21 v23.81,9.84 SV101.6 | v17.78,79.69 v17.78,58.1 v17.78,51.12 v17.78,49.53 v17.78,43.81 v17.78,38.42 v17.78,34.92 v17.78,29.84 v17.78,28.26 v17.78,22.23 v17.78,9.84 v17.78,9.21 v18.41,9.21 | v23.81,9.21 v23.18,9.21 | C201.2 51.31,93.34 C108.- | C108.- 48.13,93.98 44.13,93.98 43.5,93.34 R108.2 43.5,87.63 40.01,84.14 IC103.1 | C109.- 49.53,84.45 49.21,84.77 48.26,85.72 48.26,91.12 49.21,92.08 49.85,91.89 C108.-
  Bottom 0.61: REL202.7A v90.49,54.61 | v66.04,67.31 v53.66,67.31
  Bottom 0.813: v72.07,26.35 v63.5,26.35 | v63.5,3.81 v67.63,3.81 | IC203.17 57.15,35.88 56.2,36.83 56.2,40.01 55.24,40.96 IC203.10 | IC101.31 45.72,53.66 44.45,52.39 40.32,52.39 39.05,51.12 IC101.11 32.38,51.12 30.8,49.53 v17.78,49.53 | OK101.2 v17.78,51.12 | C104.2 C107.2 22.54,58.74 21.91,58.1 v17.78,58.1 | X101.9 17.72,43.76 v17.78,43.81 | X103.S@1 17.61,38.58 v17.78,38.42 | v17.78,22.23 17.63,22.38 X103.S@2 X102.S@1 | X103.5 7.62,30.16 | X103.4 7.81,29.97 7.62,30.16 | X103.3 7.62,30.16 | 7.62,30.16 9.21,30.16 9.53,29.84 v17.78,29.84 | X102.S@2 13.49,2.38 v13.65,2.54 | v13.65,10.16 9.59,10.16 X102.4 9.21,10.16 | 9.21,10.16 8.89,10.16 8.06,10.99 X102.5 | 9.21,10.16 17.46,10.16 v17.78,9.84 | IC104.9 29.21,24.77 28.26,25.72 20.32,25.72 v17.78,28.26 | C103.1 C102.1 C105.1 | C106.1 C105.1 | C105.1 v17.78,34.92
  Bottom 1.016: v63.5,3.81 57.15,3.81 55.56,2.22 v53.66,2.22 v40.32,2.22 v36.83,2.22 v25.08,2.22 v24.45,2.22 v23.81,2.22 v23.81,3.49 | v23.81,9.21 v23.18,9.21 v18.41,9.21 v17.78,9.21 v17.78,9.84 | v23.81,9.84 v23.81,8.57 | V101.GND 24.77,81.92 24.13,81.28 18.1,81.28 17.78,80.96 v17.78,79.69 D101.K 3.81,79.69 2.86,80.64 2.86,89.53 3.81,90.49 7.49,90.49 CON101.2 | C101.2 35.24,83.5 IC103.1
  pour Bottom: 15.24,24.77 15.24,88.27 23.81,96.84 51.75,96.84 51.75,78.74 31.43,78.74 31.43,24.77
K11
  Top 0.61: REL201.16A 68.58,92.71 67.94,92.08 67.94,82.23 71.12,79.06 71.12,75.88 72.07,74.93 REL201.9
  Bottom 0.61: REL201.9 73.98,74.93 75.25,73.66 97.47,73.66 98.42,74.61 98.42,91.44 97.47,92.39 X201.1
K12  (via drill 0.3)
  Top 0.61: v83.82,85.09 v83.82,87.31
  Bottom 0.61: REL201.13 v83.82,85.09 | v83.82,87.31 X201.2
K13  (via drill 0.3)
  Top 0.61: v85.09,81.6 v85.09,86.04 | REL201.15A 69.53,90.17 68.9,89.53 68.9,82.55 71.44,80.01 REL201.11
  Bottom 0.61: REL201.11 73.03,80.33 74.3,81.6 v85.09,81.6 | v85.09,86.04 90.81,86.04 92.71,84.14 92.71,83.19 93.66,82.23 X201.3
K21
  Top 0.61: REL202.16A 73.34,69.85 72.71,69.22 72.71,59.37 75.88,56.2 75.88,53.66 REL202.9
  Bottom 0.61: REL202.9 97.47,52.07 98.11,52.7 98.11,64.45 X202.1
K22
  Bottom 0.61: REL202.13 94.61,62.23 X202.2
K23  (via drill 0.3)
  Top 0.61: v84.45,57.15 v84.45,60.33 | REL202.15A 73.98,67.31 73.66,66.99 73.66,59.69 76.2,57.15 REL202.11
  Bottom 0.61: REL202.11 v84.45,57.15 | v84.45,60.33 93.34,60.33 94.93,58.74 X202.3
K31
  Top 0.61: REL203.16A 73.34,47.31 72.71,46.67 72.71,36.83 75.88,33.66 75.88,31.11 REL203.9
  Bottom 0.61: REL203.9 96.84,29.53 97.79,30.48 97.79,41.59 96.84,42.55 X203.1
K32  (via drill 0.3)
  Top 0.61: v88.9,39.69 v88.9,37.47
  Bottom 0.61: REL203.13 v88.9,39.69 | v88.9,37.47 X203.2
K33
  Top 0.61: REL203.15A 73.98,44.77 73.66,44.45 73.66,37.47 76.52,34.61 REL203.11
  Bottom 0.61: REL203.11 82.55,34.61 83.5,35.56 89.53,35.56 92.71,32.38 X203.3
K41
  Top 0.61: REL204.9 70.17,6.67 69.53,7.3 69.53,11.11 68.26,12.38 68.26,23.81 68.9,24.45 REL204.16A
  Bottom 0.61: REL204.9 83.5,6.67 86.04,4.13 96.84,4.13 97.79,5.08 97.79,16.51 96.84,17.46 X204.1
K42  (via drill 0.3)
  Top 0.61: v85.09,16.83 v85.09,22.86
  Bottom 0.61: REL204.13 v85.09,16.83 | v85.09,22.86 90.49,22.86 91.44,21.91 91.44,13.34 92.39,12.38 X204.2
K43
  Top 0.61: REL204.11 70.17,11.75 69.22,12.7 69.22,21.27 69.85,21.91 REL204.15A
  Bottom 0.61: REL204.11 86.68,11.75 87.95,10.48 91.76,10.48 X204.3
LED-G
  Bottom 0.406: R102.1 31.43,74.3 31.75,73.98 IC101.2
LED-R
  Bottom 0.406: R101.1 30.48,71.44 33.02,68.9 IC101.4
MISO  (via drill 0.3)
  Top 0.406: IC104.15 41.91,19.68 40.64,20.95 40.64,25.4 40.32,25.72 v40.32,61.28
  Bottom 0.406: SV101.1 22.54,15.24 26.35,15.24 27.62,13.97 41.91,13.97 | 41.91,13.97 46.67,13.97 46.99,13.65 IC102.2 | IC104.15 41.91,13.97 | v40.32,61.28 IC101.7
MOSI  (via drill 0.3)
  Top 0.406: v26.99,13.02 v26.99,10.16 | v41.91,10.16 IC102.5 | v39.37,10.16 IC104.14 39.37,19.68 38.1,20.95 38.1,25.4 38.42,25.72 v38.42,63.82
  Bottom 0.406: SV101.4 26.04,13.97 v26.99,13.02 | v26.99,10.16 v39.37,10.16 v41.91,10.16 | v38.42,63.82 IC101.6
N$1  (via drill 0.3)
  Top 0.406: IC105.1 36.83,12.7 35.56,13.97 v35.56,19.68 | v49.53,19.68 IC104.1
  Bottom 0.406: v35.56,19.68 v49.53,19.68
N$2  (via drill 0.3)
  Top 0.406: IC105.4 29.21,12.7 30.48,13.97 v30.48,18.73 | v46.99,18.73 IC104.2
  Bottom 0.406: v30.48,18.73 v46.99,18.73
N$3
  Top 0.406: OK101.3 28.57,50.48 29.84,49.21 R106.1
N$4  (via drill 0.3)
  Top 0.406: v13.34,16.19 v13.34,53.66 | v26.35,53.66 v26.35,56.52
  Bottom 0.406: X102.3 6.92,8.95 6.35,9.53 6.35,14.29 8.26,16.19 v13.34,16.19 | v13.34,53.66 OK101.1 v26.35,53.66 | v26.35,56.52 R109.2
N$5  (via drill 0.3)
  Top 0.61: v56.52,12.06 v56.52,48.58
  Bottom 0.61: LED202.A 87.63,6.03 85.09,8.57 72.39,8.57 67.63,13.34 64.14,13.34 62.87,12.06 v56.52,12.06 | v56.52,48.58 IC203.22
N$6
  Top 1.016: D102.C 28.57,87.95 27.3,86.68 V101.IN 28.57,82.55 46.04,82.55 C109.+
  Bottom 0.813: D102.C C110.1
N$7  (via drill 0.3)
  Top 0.61: LED201.A v87.95,13.34 | v55.56,14.61 v55.56,46.04
  Bottom 0.61: v87.95,13.34 69.53,13.34 68.26,14.61 v55.56,14.61 | v55.56,46.04 IC203.21
N$8  (via drill 0.3)
  Top 0.61: IC201.16 IC201.15 | REL201.15 v73.03,87 | v63.82,87 v63.82,84.14
  Bottom 0.61: v73.03,87 v63.82,87 | v63.82,84.14 IC201.16
N$9  (via drill 0.3)
  Top 0.406: v12.38,77.15 v12.38,71.44
  Bottom 0.406: D101.AR v12.38,77.15 | v12.38,71.44 R101.2
N$10  (via drill 0.3)
  Top 0.61: v57.47,42.23 v57.47,51.12
  Bottom 0.61: LED203.A 64.45,41.27 63.5,42.23 v57.47,42.23 | v57.47,51.12 IC203.23
N$11  (via drill 0.3)
  Top 0.61: v71.75,63.82 71.75,59.05 74.93,55.88 v74.93,50.16 | v59.37,49.85 59.37,55.88 59.69,56.2 IC203.25
  Bottom 0.61: LED205.A 87.95,64.45 87.31,63.82 v71.75,63.82 | v74.93,50.16 67.94,50.16 67.63,49.85 v59.37,49.85
N$12  (via drill 0.3)
  Top 0.61: v83.82,64.77 83.82,77.15 86.04,79.38 86.04,89.22 LED207.A
  Bottom 0.61: IC203.27 61.91,61.28 63.18,62.55 66.99,62.55 69.22,64.77 v83.82,64.77
N$13  (via drill 0.3)
  Top 0.406: v13.34,82.23 v13.34,74.3
  Bottom 0.406: D101.AG v13.34,82.23 | v13.34,74.3 R102.2
N$14
  Top 0.61: RN201.1 65.41,65.09 63.82,66.67 63.82,76.83 64.45,77.47 REL201.7
  Bottom 0.61: RN201.1 65.41,64.45 64.77,65.09 56.52,65.09 55.24,63.82 IC203.1
N$15  (via drill 0.3)
  Top 0.61: v56.52,57.47 v56.52,61.28
  Bottom 0.61: REL202.7 68.26,54.61 67.63,55.24 67.63,58.1 66.99,58.74 RN201.3 64.14,58.74 62.87,57.47 v56.52,57.47 | v56.52,61.28 IC203.2
N$16  (via drill 0.3)
  Top 0.61: RN201.5 66.99,53.66 67.63,54.29 67.63,58.1 68.26,58.74 70.8,58.74 73.98,55.56 73.98,50.16 71.75,47.94 v71.75,36.51 | v55.56,54.93 v55.56,58.74
  Bottom 0.61: v71.75,36.51 67.94,36.51 67.31,35.88 67.31,32.7 67.94,32.07 REL203.7 | RN201.5 64.77,53.66 63.5,54.93 v55.56,54.93 | v55.56,58.74 IC203.3
N$17  (via drill 0.3)
  Top 0.61: v58.42,9.53 v58.42,47.31 v58.42,56.2
  Bottom 0.61: REL204.7 64.14,9.21 63.82,9.53 v58.42,9.53 | v58.42,47.31 63.18,47.31 64.45,48.58 RN201.7 | v58.42,56.2 IC203.4
N$18  (via drill 0.3)
  Top 0.61: v67.31,52.39 v67.31,27.3 | v87.95,27.3 LED204.A
  Bottom 0.61: IC203.24 62.23,53.66 63.5,52.39 v67.31,52.39 | v67.31,27.3 v87.95,27.3
N$19
  Bottom 0.61: IC203.26 62.23,58.74 63.5,60.01 81.28,60.01 82.23,59.05 84.45,59.05 87.31,56.2 LED206.A
N$20  (via drill 0.3)
  Top 0.61: IC203.28 v61.28,66.36 | v66.99,66.36 66.99,71.75 67.63,72.39 80.96,72.39 81.28,72.71 v81.28,80.01
  Bottom 0.61: v61.28,66.36 v66.99,66.36 | v81.28,80.01 87,80.01 LED208.A
N$21  (via drill 0.3)
  Top 0.406: C102.2 22.23,43.69 Q101.2 | v30.48,44.45 30.48,46.99 32.07,48.58 IC101.12
  Bottom 0.406: Q101.2 22.67,44.26 23.81,45.4 27.94,45.4 28.89,44.45 v30.48,44.45
N$22  (via drill 0.3)
  Top 0.406: C103.2 27.62,44.01 Q101.1 | IC101.13 31.75,46.04 31.43,45.72 v31.43,43.5
  Bottom 0.406: v31.43,43.5 28.13,43.5 Q101.1
N$23
  Top 0.406: C105.2 22.23,28.38 Q102.2 22.54,27.81 22.54,26.67 23.5,25.72 31.43,25.72 31.75,25.4 IC104.8
N$24
  Top 0.406: C106.2 27.62,28.07 Q102.1 28.77,26.67 33.97,26.67 34.29,26.35 IC104.7
N$37
  Top 0.61: IC201.12 IC201.11
  Bottom 0.61: REL202.15 78.74,67.31 79.06,67.63 79.06,71.75 78.42,72.39 64.14,72.39 63.18,71.44 IC201.11
N$50  (via drill 0.3)
  Top 0.61: IC202.15 IC202.16 60.01,20.95 59.37,21.59 v59.37,44.77
  Bottom 0.61: REL203.15 77.47,43.5 77.15,43.18 66.36,43.18 64.77,44.77 v59.37,44.77
N$52  (via drill 0.3)
  Top 0.61: IC202.11 IC202.12 | v59.37,19.68 v59.37,10.79
  Bottom 0.61: REL204.15 73.03,20.32 72.39,19.68 v59.37,19.68 | v59.37,10.79 IC202.12
P00  (via drill 0.3)
  Top 0.406: IC201.1 IC201.2 56.83,86.68 57.47,86.04 v57.47,62.55 | v37.47,62.55 v37.47,43.5
  Bottom 0.406: v57.47,62.55 v37.47,62.55 | v37.47,43.5 IC101.14
P01  (via drill 0.3)
  Top 0.406: IC201.3 IC201.4 55.88,81.6 56.52,80.96 v56.52,66.36 | v36.51,65.09 v36.51,38.42
  Bottom 0.406: v56.52,66.36 52.39,66.36 51.12,65.09 v36.51,65.09 | v36.51,38.42 IC101.16
P02  (via drill 0.3)
  Top 0.406: IC201.5 IC201.6 | v55.56,76.52 v55.56,72.71 | v46.04,72.71 v46.04,33.34
  Bottom 0.406: IC201.6 v55.56,76.52 | v55.56,72.71 v46.04,72.71 | v46.04,33.34 IC101.18
P03  (via drill 0.3)
  Top 0.406: IC201.7 IC201.8 | v46.99,70.17 v46.99,28.26
  Bottom 0.406: IC201.8 52.39,70.17 v46.99,70.17 | v46.99,28.26 IC101.20
P04  (via drill 0.3)
  Top 0.406: IC202.2 IC202.1 53.66,27.62 51.75,29.53 v51.75,39.69 | v43.18,39.69 v43.18,48.58
  Bottom 0.406: v51.75,39.69 v43.18,39.69 | v43.18,48.58 IC101.29
P05  (via drill 0.3)
  Top 0.406: IC202.4 IC202.3 | v50.8,20.95 v50.8,37.15 | v39.37,37.15 v39.37,43.5
  Bottom 0.406: IC202.3 v50.8,20.95 | v50.8,37.15 v39.37,37.15 | v39.37,43.5 IC101.27
P06  (via drill 0.3)
  Top 0.406: IC202.6 IC202.5 | v43.18,17.78 v43.18,38.42
  Bottom 0.406: IC202.5 52.7,15.88 50.8,17.78 v43.18,17.78 | v43.18,38.42 IC101.25
P07  (via drill 0.3)
  Top 0.406: IC202.8 IC202.7 | v45.72,10.16 45.72,25.4 44.13,26.99 v44.13,66.36
  Bottom 0.406: IC202.7 52.07,10.79 51.44,10.16 v45.72,10.16 | v44.13,66.36 IC101.36
P20  (via drill 0.3)
  Top 0.406: v20.95,42.55 20.95,46.67 22.54,48.26 22.54,57.47 20.95,59.05 v20.95,69.85
  Bottom 0.406: IC101.15 31.75,40.96 30.16,42.55 v20.95,42.55 | v20.95,69.85 7.21,69.85 X101.1
P21  (via drill 0.3)
  Top 0.406: v26.04,36.2 26.04,46.04 25.4,46.67 v25.4,67.31
  Bottom 0.406: IC101.17 31.11,35.88 30.8,36.2 v26.04,36.2 | v25.4,67.31 6.25,67.31 X101.2
P22  (via drill 0.3)
  Top 0.406: v25.08,30.8 25.08,46.04 24.45,46.67 v24.45,64.14
  Bottom 0.406: IC101.19 v25.08,30.8 | v24.45,64.14 5.92,64.14 X101.3
P23  (via drill 0.3)
  Top 0.406: v24.13,29.53 24.13,46.04 23.5,46.67 v23.5,61.28
  Bottom 0.406: IC101.21 48.58,28.26 47.31,29.53 v24.13,29.53 | v23.5,61.28 5.32,61.28 X101.4
P24  (via drill 0.3)
  Top 0.406: v42.23,46.04 v42.23,38.42 | v10.48,37.15 v10.48,57.78
  Bottom 0.406: IC101.28 v42.23,46.04 | v42.23,38.42 38.1,38.42 36.83,37.15 31.43,37.15 29.84,38.73 21.27,38.73 19.68,37.15 v10.48,37.15 | v10.48,57.78 5.33,57.78 X101.5
P25  (via drill 0.3)
  Top 0.406: v20,41.59 v20,45.72 | v9.53,45.72 v9.53,54.29
  Bottom 0.406: IC101.26 36.83,40.96 35.56,39.69 31.75,39.69 29.84,41.59 v20,41.59 | v20,45.72 v9.53,45.72 | v9.53,54.29 5.33,54.29 X101.6
P26  (via drill 0.3)
  Top 0.406: v29.53,34.61 v29.53,46.99 | v8.57,46.99 v8.57,50.8
  Bottom 0.406: IC101.24 38.1,35.88 36.83,34.61 v29.53,34.61 | v29.53,46.99 v8.57,46.99 | v8.57,50.8 5.34,50.8 X101.7
P27  (via drill 0.3)
  Top 0.406: v7.62,47.31 v7.62,55.24 | v20,55.24 20.32,55.24 v21.59,56.52 | v35.56,62.55 v35.56,60.01 | v43.18,60.01 v43.18,63.82
  Bottom 0.406: X101.8 7.25,47.26 7.3,47.31 v7.62,47.31 | v7.62,55.24 v20,55.24 | v21.59,56.52 23.18,56.52 24.45,57.78 27.3,57.78 27.94,58.42 27.94,61.28 28.26,61.59 30.48,61.59 31.43,62.55 v35.56,62.55 | v35.56,60.01 v43.18,60.01 | v43.18,63.82 IC101.35
PLUGGED  (via drill 0.3)
  Top 0.406: CON101.3 10.65,72.88 v10.79,72.71
  Bottom 0.406: v10.79,72.71 42.86,72.71 44.13,73.98 IC101.39
S1  (via drill 0.3)
  Top 0.61: IC201.17 IC201.18 v61.28,94.61 | v73.03,94.61 REL201.16
  Bottom 0.61: v61.28,94.61 v73.03,94.61
S2  (via drill 0.3)
  Top 0.61: IC201.14 IC201.13 | v59.37,70.17 v59.37,76.52
  Bottom 0.61: REL202.16 77.47,71.12 77.15,71.44 64.77,71.44 63.5,70.17 v59.37,70.17 | v59.37,76.52 IC201.13
S3  (via drill 0.3)
  Top 0.61: IC202.17 IC202.18 | v57.47,26.04 v57.47,34.61 | v66.36,34.61 v66.36,42.23
  Bottom 0.61: IC202.18 v57.47,26.04 | v57.47,34.61 v66.36,34.61 | v66.36,42.23 79.06,42.23 79.69,42.86 79.69,46.67 79.06,47.31 REL203.16
S4
  Top 0.61: IC202.13 IC202.14
  Bottom 0.61: REL204.16 74.61,24.45 75.88,25.72 79.69,25.72 80.96,24.45 80.96,19.68 79.69,18.41 64.45,18.41 63.5,17.46 63.5,16.51 62.87,15.88 IC202.14
SCK  (via drill 0.3)
  Top 0.406: v26.04,12.7 v26.04,17.78 | v36.83,17.78 IC104.13 | IC104.13 36.83,19.68 35.56,20.95 35.56,58.42 35.24,58.74 IC101.8 | IC104.13 36.83,15.56 38.42,13.97 v38.42,6.35 | v44.45,6.35 IC102.6
  Bottom 0.406: SV101.3 22.54,12.7 v26.04,12.7 | v26.04,17.78 v36.83,17.78 | v38.42,6.35 v44.45,6.35
SCL
  Bottom 0.406: IC101.22 50.16,30.8 51.44,32.07 55.24,32.07 55.88,32.7 55.88,35.24 55.24,35.88 IC203.12
SDA
  Bottom 0.406: IC203.13 IC101.23
SPG
  Bottom 0.406: R107.2 R108.1 43.18,80.33 46.99,76.52 IC101.40
V-NETZTEIL
  Bottom 1.016: D103.A 21.91,93.34 19.05,90.49 13.66,90.49 CON101.1

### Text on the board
Bottom: MBCAN-Projekt | (c) Dr.-Ing. Th. Wiesner | 01.04.2024 | bottom | mbc91.brd
tNames: HW: 24.04.01 | CH 1 | STATUS | (c) Dr.-Ing. Th. Wiesner | MBCAN-Projekt | CH 2 | IN | CH 3 | OUT | CH 4 | mbc-91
